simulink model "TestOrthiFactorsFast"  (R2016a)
settings: Solver=FixedStepDiscrete  StartTime=0.0  StopTime=10  RelTol=1e-3
InitFcn:
  | Tstep=0.001;
  | %src2genBus.lib_OrthOsc_genBus();
libraries: lib_T1Blocks_FB x2, lib_OrthOsc x1, lib_AngleBlocks x1

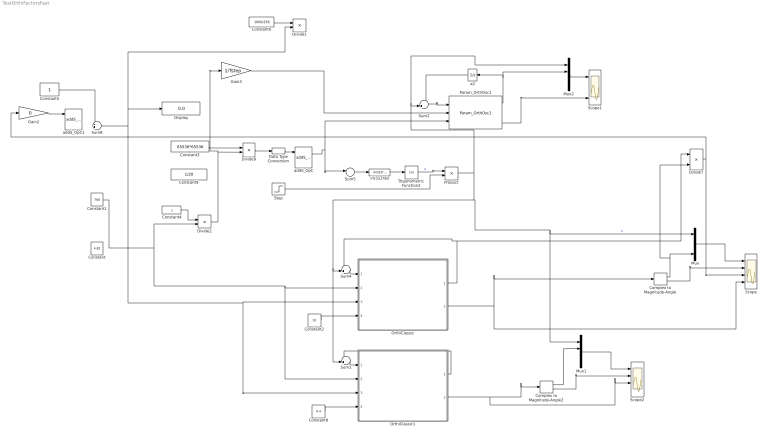
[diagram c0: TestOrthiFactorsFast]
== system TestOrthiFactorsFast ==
  Complex to Magnitude-Angle : ComplexToMagnitudeAngle
  Complex to Magnitude-Angle2 : ComplexToMagnitudeAngle
  Constant : Constant  Value=4.82  OutDataTypeStr=single
  Constant1 : Constant  Value=768  OutDataTypeStr=single
  Constant2 : Constant  Value=10  OutDataTypeStr=single
  Constant3 : Constant  Value=65536*65536  OutDataTypeStr=single
  Constant4 : Constant  OutDataTypeStr=single
  Constant5 : Constant  OutDataTypeStr=single
  Constant6 : Constant  Value=1000/256  OutDataTypeStr=single
  Constant8 : Constant  Value=0.4  OutDataTypeStr=single
  Constant9 : Constant  Value=1/20  OutDataTypeStr=single
  Data Type Conversion : DataTypeConversion  OutDataTypeStr=int32
  Display : Display
  Divide1 : Product  Inputs=**
  Divide2 : Product  Inputs=*/
  Divide7 : Product  Inputs=**/
  Divide9 : Product  Inputs=**
  Gain2 : Gain  Gain=0
  Gain3 : Gain  Gain=1/Tstep
  Mux : Mux
  Mux1 : Mux
  Mux2 : Mux  Commented=on
  OrthiClassic : Subsystem
  OrthiClassic1 : Subsystem
  Param_OrthOsc1 : lib_OrthOsc/Param_OrthOsc1  Commented=on  ident=21  Tstep=Tstep
  Product : Product
  Scope : Scope  NumInputPorts=4
  Scope1 : Scope  NumInputPorts=4
  Scope2 : Scope  NumInputPorts=4
  Step : Step  Time=1.6  Before=1  After=0.5  SampleTime=0
  Sum1 : Sum  Inputs=-+|
  Sum2 : Sum  Commented=on  Inputs=-+|
  Sum4 : Sum  Inputs=-+|
  Sum5 : Sum  Inputs=|++
  Sum8 : Sum  Inputs=++|
  Trigonometric Function2 : Trigonometry  Operator=cos
  a2 : UnitDelay  Commented=on  SampleTime=Tstep
  addS_OpC : lib_T1Blocks_FB/addS_OpC
  addS_OpC1 : lib_T1Blocks_FB/addS_OpC
  int322rad : lib_AngleBlocks/int322rad
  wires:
  Mux/1 -> Scope/1
  addS_OpC/1 -> Param_OrthOsc1/3, Sum5/1
  Constant3/1 -> Divide9/1
  int322rad/1 -> Trigonometric Function2/1
  Sum5/1 -> int322rad/1
  Trigonometric Function2/1 -> Product/1  "x"
  Complex to Magnitude-Angle/1 -> Mux/4, Divide7/3
  Complex to Magnitude-Angle/2 -> Scope/2
  Divide9/1 -> Data Type Conversion/1
  Constant1/1 -> OrthiClassic1/2(In4), OrthiClassic/2(In4), Divide2/2
  Gain2/1 -> addS_OpC1/1
  addS_OpC1/2 -> ?
  Constant5/1 -> Sum8/1
  Divide7/1 -> Scope/3, Gain2/1
  Constant6/1 -> Divide1/1
  Sum8/1 -> Display/1, Divide1/2, OrthiClassic1/3(In1), OrthiClassic/3(In1)
  OrthiClassic/1(Out6) -> Sum4/1, Divide7/1
  OrthiClassic/2(Out4) -> Complex to Magnitude-Angle/1, Scope/4
  Sum4/1 -> OrthiClassic/1(In2)
  Constant4/1 -> Divide2/1
  Divide2/1 -> Gain3/1, Divide9/2
  Constant2/1 -> OrthiClassic/4(In3)
  Sum1/1 -> OrthiClassic1/1(In2)
  OrthiClassic1/1(Out6) -> Sum1/1
  Constant8/1 -> OrthiClassic1/4(In3)
  Product/1 -> Mux2/1, Sum2/2, Mux1/1, Mux/1, Sum1/2, Sum4/2  "x"
  Mux1/1 -> Scope2/1
  ? -> Mux1/4
  Complex to Magnitude-Angle2/2 -> Scope2/2
  OrthiClassic1/2(Out4) -> Complex to Magnitude-Angle2/1, Scope2/3
  Complex to Magnitude-Angle2/1 -> Mux1/2
  Sum2/1 -> Param_OrthOsc1/1
  Param_OrthOsc1/1 -> a2/1, Mux2/2
  Gain3/1 -> Param_OrthOsc1/2
  Mux2/1 -> Scope1/1
  a2/1 -> Sum2/1
  Data Type Conversion/1 -> addS_OpC/1
  Param_OrthOsc1/4 -> Scope1/4
  Step/1 -> Product/2

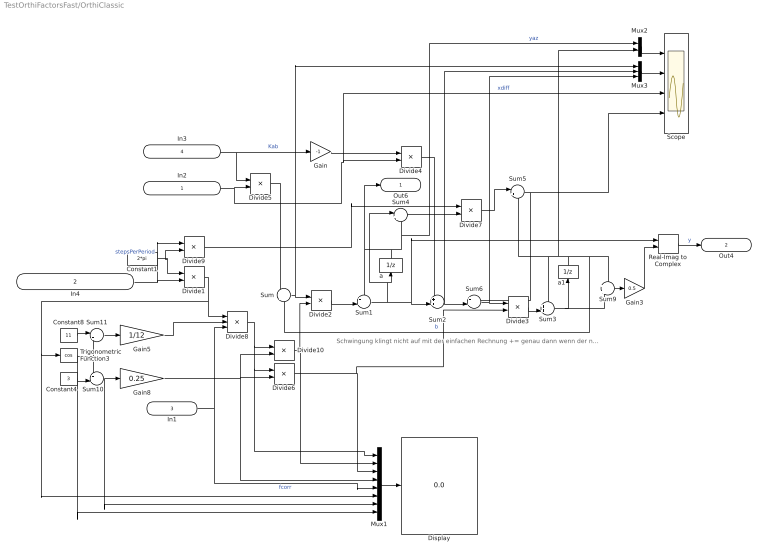
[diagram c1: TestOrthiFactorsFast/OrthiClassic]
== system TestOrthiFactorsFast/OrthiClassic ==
  note: Schwingung klingt nicht auf mit der einfachen Rechnung += genau dann wenn der neue Wert für den b-Integrator benutzt wird. Damit ist 1 Totzeit im System, neben den Integratoren. Mit 2 Totzeiten, symmetrische Schaltung, klingt die Schwingung immer auf, wenn das einfache += verwendet wird.
  In2 : Inport
  In4 : Inport  Port=2
  In1 : Inport  Port=3
  In3 : Inport  Port=4
  Constant1 : Constant  Value=2*pi  OutDataTypeStr=single
  Constant4 : Constant  Value=3  OutDataTypeStr=single
  Constant8 : Constant  Value=11  OutDataTypeStr=single
  Display : Display
  Divide1 : Product  Inputs=*/
  Divide10 : Product  Inputs=*/
  Divide{2..7} (6 alike) : Product  Inputs=**
  Divide8 : Product  Inputs=***
  Divide9 : Product  Inputs=*/
  Gain : Gain  Gain=-1
  Gain3 : Gain  Gain=0.5
  Gain5 : Gain  Gain=1/12
  Gain8 : Gain  Gain=0.25
  Mux1 : Mux  Inputs=8
  Mux2 : Mux  Inputs=2
  Mux3 : Mux  Inputs=3
  Real-Imag to Complex : RealImagToComplex
  Scope : Scope  NumInputPorts=4
  Sum : Sum  Inputs=+|-
  Sum{1..3,6,10} (5 alike) : Sum  Inputs=++|
  Sum11 : Sum  Inputs=|++
  Sum4 : Sum  Inputs=|+-
  Sum5 : Sum  Inputs=|++
  Sum9 : Sum  Inputs=+|+
  Trigonometric Function3 : Trigonometry  Operator=cos
  a : UnitDelay  InitialCondition=1  SampleTime=Tstep
  a1 : UnitDelay  SampleTime=Tstep
  Out6 : Outport
  Out4 : Outport  Port=2
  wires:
  In4/1 -> Divide9/1, Divide1/2  "stepsPerPeriod"
  Gain5/1 -> Divide8/2
  In2/1 -> Divide5/2, Scope/3, Divide4/2  "xdiff"
  Sum1/1 -> Real-Imag to Complex/1, Sum2/2, Sum4/1, a/1
  Divide2/1 -> Sum1/2
  a/1 -> Mux2/1, Sum4/2, Out6/1, Sum1/1  "yaz"
  Divide3/1 -> Sum3/2
  a1/1 -> Sum/2, Sum9/1, Sum5/2, Sum3/1, Mux2/2  "b"
  Sum/1 -> Mux3/1, Divide2/1
  Sum2/1 -> Sum6/2, Mux3/2
  Divide5/1 -> Sum/1
  Divide4/1 -> Sum2/1
  Divide10/1 -> Mux1/2, Divide2/2
  Mux1/1 -> Display/1
  In3/1 -> Gain/1, Divide5/1  "Kab"
  Gain/1 -> Divide4/1
  Sum3/1 -> Sum9/2, a1/1
  Real-Imag to Complex/1 -> Out4/1  "y"
  Divide6/1 -> Mux1/3, Divide3/2
  Divide8/1 -> Mux1/1, Divide6/1, Divide10/1
  Trigonometric Function3/1 -> Mux1/8, Sum11/2, Sum10/1
  Sum10/1 -> Mux1/7, Gain8/1
  Gain8/1 -> Mux1/4, Divide6/2, Divide10/2
  Sum9/1 -> Gain3/1
  Gain3/1 -> Real-Imag to Complex/2
  Constant8/1 -> Sum11/1
  Constant4/1 -> Sum10/2
  Sum11/1 -> Gain5/1
  In1/1 -> Divide8/3, Mux1/5  "fcorr"
  Constant1/1 -> Divide1/1, Divide9/2
  Divide1/1 -> Divide8/1, Mux1/6, Trigonometric Function3/1
  Divide7/1 -> Sum5/1
  Mux2/1 -> Scope/1
  Sum4/1 -> Divide7/2
  Divide9/1 -> Divide7/1
  Mux3/1 -> Scope/2
  Sum5/1 -> Sum6/1, Scope/4
  Sum6/1 -> Mux3/3, Divide3/1

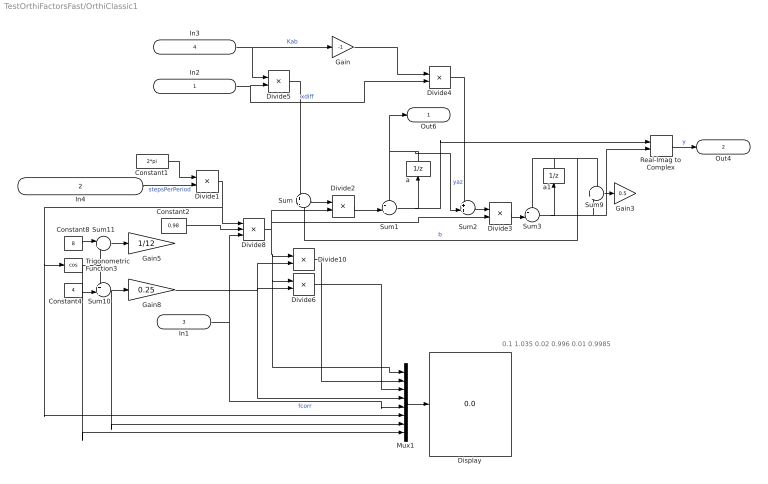
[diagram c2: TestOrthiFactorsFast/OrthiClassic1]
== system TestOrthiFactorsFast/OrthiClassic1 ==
  note: 0.1 1.035 0.02 0.996 0.01 0.9985
  In2 : Inport
  In4 : Inport  Port=2
  In1 : Inport  Port=3
  In3 : Inport  Port=4
  Constant1 : Constant  Value=2*pi  OutDataTypeStr=single
  Constant2 : Constant  Value=0.98  OutDataTypeStr=single
  Constant4 : Constant  Value=4  OutDataTypeStr=single
  Constant8 : Constant  Value=8  OutDataTypeStr=single
  Display : Display
  Divide1 : Product  Inputs=*/
  Divide10 : Product  Inputs=*/
  Divide{2..6} (5 alike) : Product  Inputs=**
  Divide8 : Product  Inputs=***
  Gain : Gain  Gain=-1
  Gain3 : Gain  Gain=0.5
  Gain5 : Gain  Gain=1/12
  Gain8 : Gain  Gain=0.25
  Mux1 : Mux  Inputs=8
  Real-Imag to Complex : RealImagToComplex
  Sum : Sum  Inputs=+|-
  Sum{1..3,10} (4 alike) : Sum  Inputs=++|
  Sum11 : Sum  Inputs=|++
  Sum9 : Sum  Inputs=+|+
  Trigonometric Function3 : Trigonometry  Operator=cos
  a : UnitDelay  InitialCondition=1  SampleTime=Tstep
  a1 : UnitDelay  SampleTime=Tstep
  Out6 : Outport
  Out4 : Outport  Port=2
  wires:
  In4/1 -> Divide1/2  "stepsPerPeriod"
  Gain5/1 -> ?
  In2/1 -> Divide5/2, Divide4/2  "xdiff"
  Sum1/1 -> Real-Imag to Complex/1, a/1
  Divide2/1 -> Sum1/2
  a/1 -> Sum2/2, Out6/1, Sum1/1  "yaz"
  Divide3/1 -> Sum3/2
  a1/1 -> Sum/2, Sum9/1, Sum3/1  "b"
  Sum/1 -> Divide2/1
  Sum2/1 -> Divide3/1
  Divide5/1 -> Sum/1
  Divide4/1 -> Sum2/1
  Divide10/1 -> Mux1/2
  Mux1/1 -> Display/1
  In3/1 -> Gain/1, Divide5/1  "Kab"
  Gain/1 -> Divide4/1
  Sum3/1 -> Real-Imag to Complex/2, Sum9/2, a1/1
  Real-Imag to Complex/1 -> Out4/1  "y"
  Divide6/1 -> Mux1/3
  Divide8/1 -> Divide3/2, Divide2/2, Mux1/1, Divide6/1, Divide10/1
  Trigonometric Function3/1 -> Mux1/8, Sum11/2, Sum10/1
  Sum10/1 -> Mux1/7, Gain8/1
  Gain8/1 -> Mux1/4, Divide6/2, Divide10/2
  Sum9/1 -> Gain3/1
  Constant8/1 -> Sum11/1
  Constant4/1 -> Sum10/2
  Sum11/1 -> Gain5/1
  In1/1 -> Divide8/3, Mux1/5  "fcorr"
  Constant1/1 -> Divide1/1
  Divide1/1 -> Divide8/1, Mux1/6, Trigonometric Function3/1
  Constant2/1 -> Divide8/2
